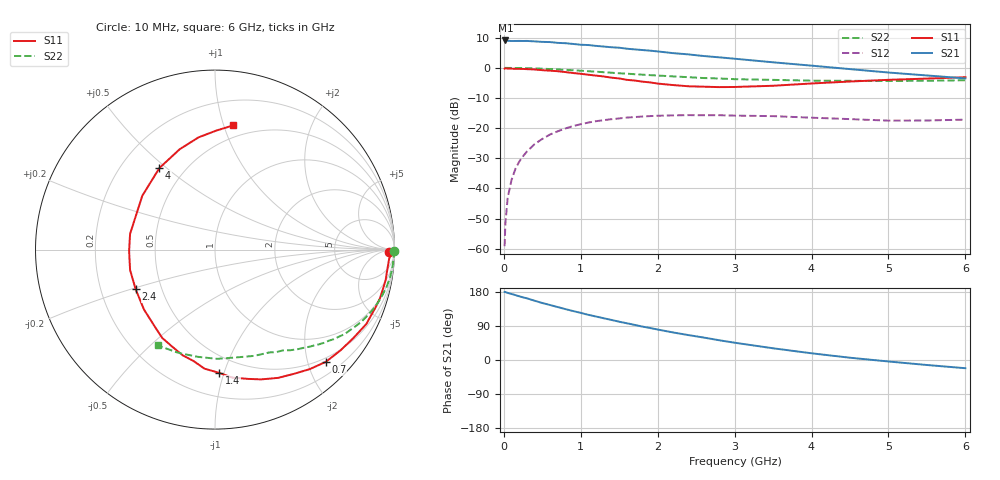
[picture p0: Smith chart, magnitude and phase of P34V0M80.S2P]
! SIEMENS Small Signal Semiconductors
! BFP181
! Si NPN RF Bipolar Junction Transistor in SOT143
! VCE = 4 V  IC = 0.8 mA
! Common Emitter S-Parameters:  March  1996
# GHz  S  MA  R  50
!  f  S11  S21  S12  S22
! GHz  MAG  ANG  MAG  ANG  MAG  ANG  MAG  ANG
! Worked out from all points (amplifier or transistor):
!   36 points, 10 MHz to 6 GHz, reference 50 ohm
!   highest |S21| = 9.1 dB at 20 MHz (marker M1)
!   |S21| within 3 dB of that: start of sweep to 1.718 GHz
!   unconditionally stable (mu >= 1): 3.391 GHz to end of sweep
!   at 250 MHz: K = 0.08, MSG = 19.1 dB, |S12| = -29.3 dB
!   at 1.4 GHz: K = 0.46, MSG = 11.9 dB, |S12| = -17.0 dB
!   at 6 GHz: K = 1.32, MAG = 3.4 dB, |S12| = -17.2 dB
!   S11 on the Smith chart (normalised r, x): 10 MHz: 54, -25; 700 MHz: 0.42, -2.33; 1.4 GHz: 0.37, -0.96; 2.4 GHz: 0.36, -0.21; 4 GHz: 0.36, +0.47; 6 GHz: 0.40, +1.08
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0.01  0.9699 -0.8  2.82 179.6  0.0011 90.9  0.9989 -0.3
0.02  0.9827 -1.6  2.845 179.4  0.0026 90.3  0.998 -0.6
0.05  0.9719 -2.9  2.81 177.0  0.007 90.3  0.9969 -1.6
0.1  0.9665 -6.7  2.786 174.2  0.0138 84.4  0.9954 -3.1
0.2  0.9612 -13.2  2.795 168.1  0.0278 81.5  0.9929 -6.2
0.3  0.951 -19.7  2.795 162.8  0.0409 76.6  0.9867 -9.2
0.5  0.9146 -32.7  2.695 150.4  0.0662 67.9  0.9671 -15.1
0.6  0.8964 -38.9  2.675 145.1  0.0783 63.4  0.9546 -18.1
0.7  0.8791 -45.3  2.594 139.7  0.0885 59.7  0.9406 -20.8
0.8  0.8503 -51.5  2.562 134.3  0.0987 55.7  0.9258 -23.4
1.1  0.7676 -70.4  2.387 119.1  0.1238 44.9  0.8782 -30.5
1.4  0.6869 -88.1  2.192 105.7  0.1406 35.0  0.8292 -37.0
1.5  0.6661 -95.0  2.157 101.0  0.1448 32.5  0.8119 -38.7
1.8  0.59 -114.1  1.973 88.2  0.1556 25.2  0.7701 -43.8
2.2  0.5178 -139.8  1.752 72.7  0.1626 16.3  0.7213 -50.3
2.4  0.4943 -153.4  1.671 65.7  0.164 12.4  0.6995 -53.3
3  0.4812 169.5  1.416 45.6  0.1613 3.3  0.6481 -62.1
3.5  0.504 143.5  1.235 30.9  0.1579 -2.0  0.6312 -69.7
4  0.5502 124.2  1.087 17.7  0.1489 -5.5  0.6125 -78.7
4.5  0.5927 109.4  0.952 6.0  0.141 -7.9  0.6088 -88.9
5.5  0.6634 89.3  0.747 -13.2  0.1337 -3.7  0.6105 -109.9
6  0.6992 81.7  0.668 -21.7  0.1383 -1.8  0.6221 -120.9
